| TEXAS INSTRUMENTS INCORPORATED
| Standard Linear and Logic Group
| IBIS Model of SN74CB3Q3251
| 2.5-V/3.3-V LOW-VOLTAGE HIGH-BANDWIDTH 1-OF-8 FET MULTIPLEXER/DEMULTIPLEXER
| This file contains package information for the following:
|  QSOP 16-pin (DBQ) package as [Component] CB3Q3251_DBQ
|  TVSOP 16-pin (DGV) package as [Component] CB3Q3251_DGV
|  TSSOP 16-pin (PW) package as [Component] CB3Q3251_PW
| This device can be powered at the following Vccs:
|  3.3 volt Vcc
|  2.5 volt Vcc
| This file provides unique models under the [Model Selector] for each Vcc.
| For operation at a specific Vcc, select the appropriate model after each
| [Model Selector] keyword.
[IBIS Ver]   3.2
[Comment char]  |_char
[File Name]   sn74cb3q3251.ibs
[File Rev]   1.1 | b_die
[Date]   May 29, 2004
[Source]   Data create from TI-SPICE simulations at TI-SLL.
[Notes]   The following is an IBIS list for the SN74CB3Q3251.
   Please contact sllibis@ti.com with questions and
   comments concerning SLL IBIS models.
   - FILE REV HISTORY
   - 1.1 Release IBIS file on 06/02/04
   - C_comp values are taken at a different test condition than
   the Ci/Cio in data sheet.
   - Power-clamp data has been deleted since there is no
   power-clamp diode in the device.
[Disclaimer] Property of Texas Instruments Incorporated. Unauthorized
   reproduction and/or distribution is strictly prohibited.
   This product is protected under copyright law.
   Created 2002,(C) Copyright 2002, Texas Instruments
   Incorporated, All Rights Reserved
   UNLESS THERE IS A SIGNED, WRITTEN AGREEMENT TO THE
   CONTRARY, TEXAS INSTRUMENTS (TI) IS PROVIDING THE IBIS
   MODELS  AND WITHOUT ANY WARRANTY, EXPRESSED OR
   IMPLIED.  TI assumes no liability for:
   1) the accuracy of the IBIS models provided to your
   company;
   2) the proper functioning of these IBIS Models in your
   design or for any resulting applications; or
   3) infringement of patents, copyrights or intellectual
   property rights resulting from your use of these IBIS
   models.
   TI provides IBIS Models as a service to our customers.
   You and your company shall not distribute, sell or give
   these models to anyone else without prior written
   permission from TI.
   TI reserves the right to make changes to our products or
   to discontinue any semiconductor product or service
   without notice, and advises our customers to obtain the
   latest version of relevant information to verify, before
   placing orders, that the information being relied on is
   current.
   Please be aware that your receipt and use of the IBIS
   information provided shall serve as acceptance of these
   terms and conditions. If you do not accept these terms,
   you should return or destroy the IBIS models and any
   other accompanying information immediately.
| Component CB3Q3251_DBQ 16-pin QSOP
[Component]   CB3Q3251_DBQ
[Manufacturer]   Texas Instruments, Inc.
[Package]
|   typ   min   max
R_pkg   3.800e-02   2.700e-02   5.900e-02
L_pkg   2.353e-09   1.491e-09   4.500e-09
C_pkg   2.100e-13   6.400e-14   5.920e-13
[Pin]   signal_name   model_name   R_pin   L_pin   C_pin
1   B4   CB3Q3251_IOB   5.800e-02   4.450e-09   5.920e-13
2   B3   CB3Q3251_IOB   4.000e-02   1.930e-09   1.110e-13
3   B2   CB3Q3251_IOB   2.800e-02   1.538e-09   7.600e-14
4   B1   CB3Q3251_IOB   2.700e-02   1.491e-09   6.400e-14
5   A   CB3Q3251_IOA   2.700e-02   1.491e-09   6.400e-14
6   NC   NC   2.700e-02   1.506e-09   7.500e-14
7   NOE   CB3Q3251_IN   3.300e-02   1.922e-09   1.090e-13
8   GND   GND   5.900e-02   4.500e-09   5.880e-13
9   S2   CB3Q3251_IN   5.800e-02   3.695e-09   4.140e-13
10   S1   CB3Q3251_IN   3.400e-02   2.685e-09   2.820e-13
11   S0   CB3Q3251_IN   2.900e-02   1.552e-09   7.700e-14
12   B8   CB3Q3251_IOB   2.800e-02   1.506e-09   6.500e-14
13   B7   CB3Q3251_IOB   2.700e-02   1.492e-09   6.400e-14
14   B6   CB3Q3251_IOB   2.800e-02   1.534e-09   7.600e-14
15   B5   CB3Q3251_IOB   4.000e-02   2.703e-09   2.840e-13
16   VCC   POWER   5.600e-02   3.645e-09   4.180e-13
| Component CB3Q3251_DGV 16-pin TVSOP
[Component]   CB3Q3251_DGV
[Manufacturer]   Texas Instruments, Inc.
[Package]
|   typ   min   max
R_pkg   3.900e-02   3.300e-02   4.500e-02
L_pkg   2.543e-09   2.320e-09   2.938e-09
C_pkg   3.860e-13   3.340e-13   4.490e-13
[Pin]   signal_name   model_name   R_pin   L_pin   C_pin
1   B4   CB3Q3251_IOB   3.500e-02   2.907e-09   4.170e-13
2   B3   CB3Q3251_IOB   4.200e-02   2.558e-09   4.460e-13
3   B2   CB3Q3251_IOB   3.800e-02   2.341e-09   3.450e-13
4   B1   CB3Q3251_IOB   3.800e-02   2.320e-09   3.340e-13
5   A   CB3Q3251_IOA   3.900e-02   2.322e-09   3.340e-13
6   NC   NC   3.800e-02   2.353e-09   3.420e-13
7   NOE   CB3Q3251_IN   4.000e-02   2.536e-09   4.410e-13
8   GND   GND   3.300e-02   2.897e-09   4.180e-13
9   S2   CB3Q3251_IN   3.500e-02   2.927e-09   4.190e-13
10   S1   CB3Q3251_IN   4.500e-02   2.632e-09   4.490e-13
11   S0   CB3Q3251_IN   3.900e-02   2.368e-09   3.470e-13
12   B8   CB3Q3251_IOB   3.900e-02   2.330e-09   3.350e-13
13   B7   CB3Q3251_IOB   3.900e-02   2.320e-09   3.350e-13
14   B6   CB3Q3251_IOB   3.900e-02   2.361e-09   3.450e-13
15   B5   CB3Q3251_IOB   4.100e-02   2.573e-09   4.460e-13
16   VCC   POWER   3.500e-02   2.938e-09   4.200e-13
| Component CB3Q3251_PW 16-pin TSSOP
[Component]   CB3Q3251_PW
[Manufacturer]   Texas Instruments, Inc.
[Package]
|   typ   min   max
R_pkg   4.500e-02   3.800e-02   5.100e-02
L_pkg   2.593e-09   2.447e-09   3.080e-09
C_pkg   2.810e-13   2.430e-13   3.770e-13
[Pin]   signal_name   model_name   R_pin   L_pin   C_pin
1   B4   CB3Q3251_IOB   4.000e-02   3.080e-09   3.770e-13
2   B3   CB3Q3251_IOB   3.800e-02   2.458e-09   2.810e-13
3   B2   CB3Q3251_IOB   5.100e-02   2.512e-09   2.550e-13
4   B1   CB3Q3251_IOB   5.100e-02   2.447e-09   2.430e-13
5   A   CB3Q3251_IOA   5.100e-02   2.447e-09   2.430e-13
6   NC   NC   5.100e-02   2.512e-09   2.550e-13
7   NOE   CB3Q3251_IN   3.800e-02   2.458e-09   2.810e-13
8   GND   GND   4.000e-02   3.080e-09   3.770e-13
9   S2   CB3Q3251_IN   3.900e-02   2.832e-09   3.160e-13
10   S1   CB3Q3251_IN   3.800e-02   2.460e-09   2.790e-13
11   S0   CB3Q3251_IN   5.100e-02   2.512e-09   2.550e-13
12   B8   CB3Q3251_IOB   5.100e-02   2.447e-09   2.430e-13
13   B7   CB3Q3251_IOB   5.100e-02   2.447e-09   2.430e-13
14   B6   CB3Q3251_IOB   5.100e-02   2.512e-09   2.550e-13
15   B5   CB3Q3251_IOB   3.800e-02   2.459e-09   2.790e-13
16   VCC   POWER   3.900e-02   2.832e-09   3.160e-13
[Series Switch Groups]
| Function Group States
On  1 /   | A->B1 NOE LOW S0 LOW S1 LOW S2 LOW
On  2 /   | A->B2 NOE LOW S0 HIGH S1 LOW S2 LOW
On  3 /   | A->B3 NOE LOW S0 LOW S1 HIGH S2 LOW
On  4 /   | A->B4 NOE LOW S0 HIGH S1 HIGH S2 LOW
On  5 /   | A->B5 NOE LOW S0 LOW S1 LOW S2 HIGH
On  6 /   | A->B6 NOE LOW S0 HIGH S1 LOW S2 HIGH
On  7 /   | A->B7 NOE LOW S0 LOW S1 HIGH S2 HIGH
On  8 /   | A->B8 NOE LOW S0 HIGH S1 HIGH S2 HIGH
Off 1 2 3 4 5 6 7 8 /  | NOE HIGH
[Series Pin Mapping]   pin_2   model_name   function_table_group
5   4   CB3Q3251_IOA_33_S   1
| 5   4   CB3Q3251_IOA_25_S   1
5   3   CB3Q3251_IOA_33_S   2
| 5   3   CB3Q3251_IOA_25_S   2
5   2   CB3Q3251_IOA_33_S   3
| 5   2   CB3Q3251_IOA_25_S   3
5   1   CB3Q3251_IOA_33_S   4
| 5   1   CB3Q3251_IOA_25_S   4
5   15   CB3Q3251_IOA_33_S   5
| 5   15   CB3Q3251_IOA_25_S   5
5   14   CB3Q3251_IOA_33_S   6
| 5   14   CB3Q3251_IOA_25_S   6
5   13   CB3Q3251_IOA_33_S   7
| 5   13   CB3Q3251_IOA_25_S   7
5   12   CB3Q3251_IOA_33_S   8
| 5   12   CB3Q3251_IOA_25_S   8
| Model CB3Q3251_IN
[Model Selector]   CB3Q3251_IN
CB3Q3251_IN_33   3.3 volt Vcc
CB3Q3251_IN_25   2.5 volt Vcc
| Model CB3Q3251_IOA
[Model Selector]   CB3Q3251_IOA
CB3Q3251_IOA_33   3.3 volt Vcc
CB3Q3251_IOA_25   2.5 volt Vcc
| Model CB3Q3251_IOB
[Model Selector]   CB3Q3251_IOB
CB3Q3251_IOB_33   3.3 volt Vcc
CB3Q3251_IOB_25   2.5 volt Vcc
| Model CB3Q3251_IOB_S
[Model Selector]   CB3Q3251_IOB_S
CB3Q3251_IOB_33_S   3.3 volt Vcc
CB3Q3251_IOB_25_S   2.5 volt Vcc
| Model CB3Q3251_IOA_S
[Model Selector]   CB3Q3251_IOA_S
CB3Q3251_IOA_33_S   3.3 volt Vcc
CB3Q3251_IOA_25_S   2.5 volt Vcc
[Model]   CB3Q3251_IOA_33_S
Model_type  Series_switch
| variable   typ   min   max
C_comp   0   0   0
[Temperature Range]   40   100   -40
| Ambient temperature   25   85   -40
[Voltage range]   3.3   3   3.6
[On]
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[Off]
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[Model]   CB3Q3251_IOA_25_S
Model_type  Series_switch
| variable   typ   min   max
C_comp   0   0   0
[Temperature Range]   40   100   -40
| Ambient temperature   25   85   -40
[Voltage range]   2.5   2.3   2.7
[On]
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[Off]
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[Model]   CB3Q3251_IOB_33_S
Model_type  Series_switch
| variable   typ   min   max
C_comp   0   0   0
[Temperature Range]   40   100   -40
| Ambient temperature   25   85   -40
[Voltage range]   3.3   3   3.6
[On]
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[Off]
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[Model]   CB3Q3251_IOB_25_S
Model_type  Series_switch
| variable   typ   min   max
C_comp   0   0   0
[Temperature Range]   40   100   -40
| Ambient temperature   25   85   -40
[Voltage range]   2.5   2.3   2.7
[On]
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[Off]
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| Models and submodels in the file (10): CB3Q3251_IN_33 (Input), CB3Q3251_IN_25 (Input), CB3Q3251_IOA_33_S (Series_switch), CB3Q3251_IOA_33 (Terminator), CB3Q3251_IOA_25_S (Series_switch), CB3Q3251_IOA_25 (Terminator), CB3Q3251_IOB_33_S (Series_switch), CB3Q3251_IOB_33 (Terminator), CB3Q3251_IOB_25_S (Series_switch), CB3Q3251_IOB_25 (Terminator)
